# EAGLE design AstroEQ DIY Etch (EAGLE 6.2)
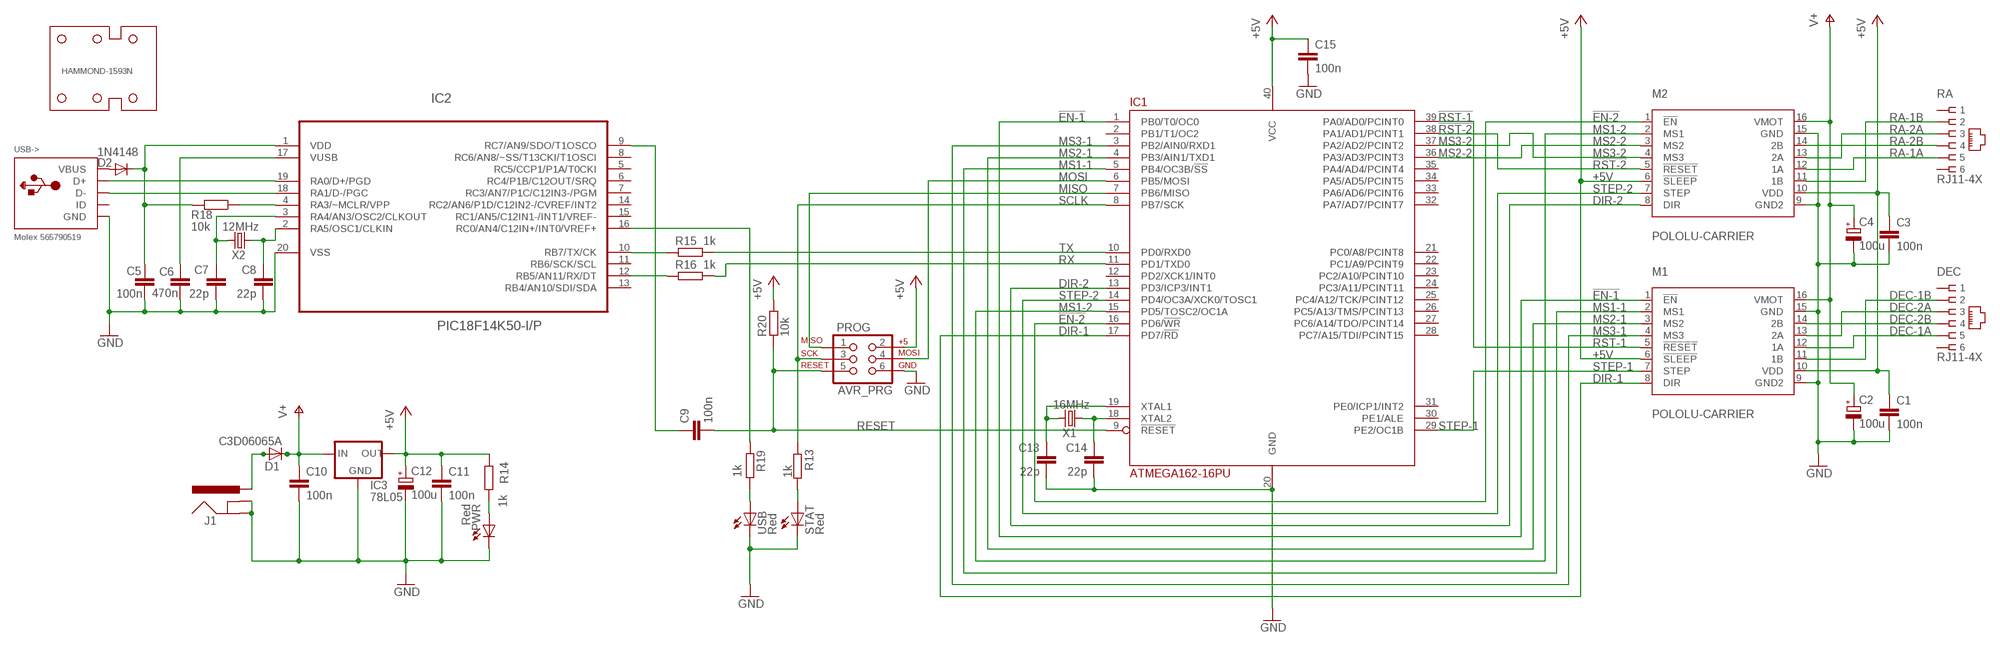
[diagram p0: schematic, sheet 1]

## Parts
C1  100n  C-EU025-024X044  [C025-024X044]
C2  100u  CPOL-EUE2.5-7  [E2,5-7]
C3  100n  C-EU025-024X044  [C025-024X044]
C4  100u  CPOL-EUE2.5-7  [E2,5-7]
C5  100n  C-EU025-024X044  [C025-024X044]
C6  470n  C-EU025-024X044  [C025-024X044]
C7  22p  C-EU025-024X044  [C025-024X044]
C8  22p  C-EU025-024X044  [C025-024X044]
C9  100n  C-EU025-024X044  [C025-024X044]
C10  100n  C-EU025-024X044  [C025-024X044]
C11  100n  C-EU025-024X044  [C025-024X044]
C12  100u  CPOL-EUE2.5-7  [E2,5-7]
C13  22p  C-EU025-024X044  [C025-024X044]
C14  22p  C-EU025-024X044  [C025-024X044]
C15  100n  C-EU025-024X044  [C025-024X044]
D1  C3D06065A  MUR820  [C221B1A]
D2  1N4148  DIODE1N4148  [DIODE-1N4148]
DEC  RJ11-4X  [RJ11-NO_SHIELD]
HAMMOND-1593N  HAMMOND-1593N  [HAMMOND-1593N]
IC1  ATMEGA162-16PU  [DIL40]
IC2  PIC18F14K50-I/P  [DIL20]
IC3  78L05  V_REG_78XXTO-92  [TO-92]
J1  POWER_JACKPTH  [POWER_JACK_PTH]
M1  POLOLU-CARRIER  A4983CARRIER  [DIP16-W]
M2  POLOLU-CARRIER  A4983CARRIER  [DIP16-W]
PROG  AVR_PRG  AVR_SPI_PRG_6PTH  [2X3]
PWR  Red  LED3MM  [LED3MM]
R13  1k  R-EU_0204/7  [0204/7]
R14  1k  R-EU_0204/7  [0204/7]
R15  1k  R-EU_0204/7  [0204/7]
R16  1k  R-EU_0204/7  [0204/7]
R18  10k  R-EU_0204/7  [0204/7]
R19  1k  R-EU_0204/7  [0204/7]
R20  10k  R-EU_0204/7  [0204/7]
RA  RJ11-4X  [RJ11-NO_SHIELD]
STAT  Red  LED3MM  [LED3MM]
USB  Red  LED3MM  [LED3MM]
USB->  Molex 565790519  USBMOLEX  [USB-MINIB-THM-MOLEX]
X1  16MHz  CRYSTALHC49US  [HC49US]
X2  12MHz  CRYSTALHC49US  [HC49US]

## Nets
!EN-1: IC1.1(PB0/T0/OC0) M1.1(!EN)
!EN-2: IC1.16(PD6/!WR) M2.1(!EN)
!RST-1: IC1.39(PA0/AD0/PCINT0) M1.5(!RESET)
!RST-2: IC1.38(PA1/AD1/PCINT1) M2.5(!RESET)
+5V: C1.1 C3.1 C11.1 C12.+ C15.1 IC1.40(VCC) IC3.1(OUT) M1.6(!SLEEP) M1.10(VDD) M2.6(!SLEEP) M2.10(VDD) PROG.2 R14.1 R20.2
AVROSC1: C13.1 IC1.19(XTAL1) X1.2
AVROSC2: C14.1 IC1.18(XTAL2) X1.1
D+: IC2.19(RA0/D+/PGD) USB->.D+
D-: IC2.18(RA1/D-/PGC) USB->.D-
DEC-1A: DEC.5 M1.12(1A)
DEC-1B: DEC.2 M1.11(1B)
DEC-2A: DEC.3 M1.13(2A)
DEC-2B: DEC.4 M1.14(2B)
DIR-1: IC1.17(PD7/!RD) M1.8(DIR)
DIR-2: IC1.13(PD3/ICP3/INT1) M2.8(DIR)
DTR: C9.1 IC2.9(RC7/AN9/SDO/T1OSCO)
GND: C1.2 C2.- C3.2 C4.- C5.2 C6.1 C7.2 C8.2 C10.2 C11.2 C12.- C13.2 C14.2 C15.2 IC1.20(GND) IC2.20(VSS) IC3.2(GND) J1.GND J1.GNDBREAK M1.9(GND2) M1.15(GND) M2.9(GND2) M2.15(GND) PROG.6 PWR.K(C) STAT.K(C) USB->.GND USB->.GND1(GND) USB->.GND4(GND) USB.K(C)
MCLR: IC2.4(RA3/~MCLR/VPP) R18.1
MISO: IC1.7(PB6/MISO) PROG.1
MOSI: IC1.6(PB5/MOSI) PROG.4
MS1-1: IC1.5(PB4/OC3B/!SS) M1.2(MS1)
MS1-2: IC1.15(PD5/TOSC2/OC1A) M2.2(MS1)
MS2-1: IC1.4(PB3/AIN1/TXD1) M1.3(MS2)
MS2-2: IC1.36(PA3/AD3/PCINT3) M2.3(MS2)
MS3-1: IC1.3(PB2/AIN0/RXD1) M1.4(MS3)
MS3-2: IC1.37(PA2/AD2/PCINT2) M2.4(MS3)
PWRLED: PWR.A R14.2
RA-1A: M2.12(1A) RA.5
RA-1B: M2.11(1B) RA.2
RA-2A: M2.13(2A) RA.3
RA-2B: M2.14(2B) RA.4
RESET: C9.2 IC1.9(!RESET) PROG.5 R20.1
RX: IC1.11(PD1/TXD0) R16.1
RX(USB): IC2.12(RB5/AN11/RX/DT) R16.2
SCLK: IC1.8(PB7/SCK) PROG.3 R13.1
STATLED: R13.2 STAT.A
STEP-1: IC1.29(PE2/OC1B) M1.7(STEP)
STEP-2: IC1.14(PD4/OC3A/XCK0/TOSC1) M2.7(STEP)
TX: IC1.10(PD0/RXD0) R15.1
TX(USB): IC2.10(RB7/TX/CK) R15.2
USBLED: R19.1 USB.A
USBOSC1: C8.1 IC2.2(RA5/OSC1/CLKIN) X2.1
USBOSC2: C7.1 IC2.3(RA4/AN3/OSC2/CLKOUT) X2.2
USBSTAT: IC2.16(RC0/AN4/C12IN+/INT0/VREF+) R19.2
V+: C2.+ C4.+ C10.1 D1.C IC3.3(IN) M1.16(VMOT) M2.16(VMOT)
VBUS: D2.A USB->.VBUS
VIN: D1.A J1.PWR
VPIC: C5.1 D2.C IC2.1(VDD) R18.2
VUSB: C6.2 IC2.17(VUSB)
Unconnected: DEC.1 DEC.6 IC1.2(PB1/T1/OC2) IC1.12(PD2/XCK1/INT0) IC1.21(PC0/A8/PCINT8) IC1.22(PC1/A9/PCINT9) IC1.23(PC2/A10/PCINT10) IC1.24(PC3/A11/PCINT11) IC1.25(PC4/A12/TCK/PCINT12) IC1.26(PC5/A13/TMS/PCINT13) IC1.27(PC6/A14/TDO/PCINT14) IC1.28(PC7/A15/TDI/PCINT15) IC1.30(PE1/ALE) IC1.31(PE0/ICP1/INT2) IC1.32(PA7/AD7/PCINT7) IC1.33(PA6/AD6/PCINT6) IC1.34(PA5/AD5/PCINT5) IC1.35(PA4/AD4/PCINT4) IC2.5(RC5/CCP1/P1A/T0CKI) IC2.6(RC4/P1B/C12OUT/SRQ) IC2.7(RC3/AN7/P1C/C12IN3-/PGM) IC2.8(RC6/AN8/~SS/T13CKI/T1OSCI) IC2.11(RB6/SCK/SCL) IC2.13(RB4/AN10/SDI/SDA) IC2.14(RC2/AN6/P1D/C12IN2-/CVREF/INT2) IC2.15(RC1/AN5/C12IN1-/INT1/VREF-) RA.1 RA.6 USB->.ID

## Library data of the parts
C1 C3 C5 C9-C11 C15 = resistor:C-EU: CAPACITOR, European symbol; MF: AVX; MPN: SR205C104KAR; OC_FARNELL: 1100367
C2 C4 C12 = resistor:CPOL-EU: POLARIZED CAPACITOR, European symbol; MF: MULTICOMP; MPN: MCGPR25V107M6.3X11; OC_FARNELL: 9451188
C6 = rcl:C-EU: CAPACITOR, European symbol; MF: KEMET; MPN: C320C474M5U5TA; OC_FARNELL: 1457660
C7 C8 C13 C14 = rcl:C-EU: CAPACITOR, European symbol; MF: AVX; MPN: SR151A220JAR; OC_FARNELL: 1100369
D1 = diode:MUR820: DIODE; MF: CREE; MPN: C3D06065A; OC_FARNELL: 1864928
D2 = SparkFun:DIODE: Diode; MF: MULTICOMP; MPN: 1N4148.; OC_FARNELL: 9565124
DEC RA = con-tycoelectronics:RJ11: CORCOM Modular RJ Jacks No Shield Source: www.tycoelectronics.com .. ENG_DS_1654001_1099_RJ_L_0507.pdf; MF: MOLEX; MPN: 95501-2641; OC_FARNELL: 1560166; OC_NEWARK: 19R7022
HAMMOND-1593N = holes:HAMMOND-1593N; MF: HAMMOND; MPN: 1593NBK; OC_FARNELL: 9287566
IC1 = atmel:ATMEGA162: 8-bit RISC MICROCONTROLLER 16K Bytes internal flash program memory 1K Bytes internal SRAM Upto 64K Bytes optional external memory space 512 Bytes EEPROM Two 8-bit timers Two 16-bit timers Dual programmable serial USARTs Master/Slave serial SPI interface Source: ATMEGA162_DIP40.lbr; MF: ATMEL; MPN: ATMEGA162-16PU; OC_FARNELL: 9171169
IC2 = microchip:PIC18F14K50-I/P: USB Flash Microcontrollers; MF: MICROCHIP; MPN: PIC18F14K50-I/P; OC_FARNELL: 1648501; OC_NEWARK: 77M3103; PACKAGE: DIP-20; SUPPLIER: Microchip
IC3 = SparkFun:V_REG_78XX: Voltage Regulator Standard 7805 5V regulator. IGO (Input Ground Output). Spark Fun Electronics SKU : COM-00107; MF: FAIRCHILD SEMICONDUCTOR; MPN: LM78L05ACZX; OC_FARNELL: 1467367
J1 = SparkFun:POWER_JACK: Power Jack This is the standard 5.5mm barrel jack for power. The PTH is the most common, proven, reliable, footprint. All others are experimental. The Slot footprint only works if the mill layer is transmitted to the PCB fab house so be warned. Spark Fun Electronics SKU : PRT-00119. Mating wall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; MF: MULTICOMP; MPN: MJ-179PH; OC_FARNELL: 1737246
M1 M2 = A4983Carrier:A4983CARRIER; MF: SAMTEC; MPN: CES-116-01-T-S; OC_FARNELL: 1667522
PROG = SparkFun:AVR_SPI_PRG_6: AVR ISP 6 Pin This is the reduced ISP connector for AVR programming. Common on Arduino. This footprint will take up less PCB space and can be used with a 10-pin to 6-pin adapter such as SKU: BOB-08508; MF: TE CONNECTIVITY / AMP; MPN: 826632-3; OC_FARNELL: 3418492
PWR STAT USB = led:LED: LED; MF: KINGBRIGHT; MPN: L-424HDT; OC_FARNELL: 1142499
R13 R14 R19 = rcl:R-EU_: RESISTOR, European symbol; MF: MULTICOMP; MPN: MF12 1K; OC_FARNELL: 9342400
R15 R16 = SmartPrj:R-EU_: RESISTOR, European symbol; MF: MULTICOMP; MPN: MF12 1K; OC_FARNELL: 9342400
R18 R20 = rcl:R-EU_: RESISTOR, European symbol; MF: MULTICOMP; MPN: MF12 10K; OC_FARNELL: 9342419
USB-> = adafruit:USB: USB Connectors USBMINIB - Surface Mount Female Mini-B USB Connector 4UConnector: 06564 By microbuilder.eu Thru-hole RA Female Mini-B USB Connector 4UConnector: 18732 By ladyada.net; MF: MOLEX; MPN: 565790519; OC_FARNELL: 1125347
X1 = SparkFun:CRYSTAL: Crystals; MF: TXC; MPN: 9B-16.000MEEJ-B; OC_FARNELL: 1842217
X2 = SparkFun:CRYSTAL: Crystals; MF: TXC; MPN: 9B-12.000MAAJ-B; OC_FARNELL: 1842203

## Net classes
1 power: width 0.61 mm, drill 0.711 mm, clearance 0.203 mm
2 gnd: width 0.305 mm, drill 0.711 mm, clearance 0.203 mm
3 usbvcc: width 0.508 mm, drill 0.711 mm, clearance 0.203 mm

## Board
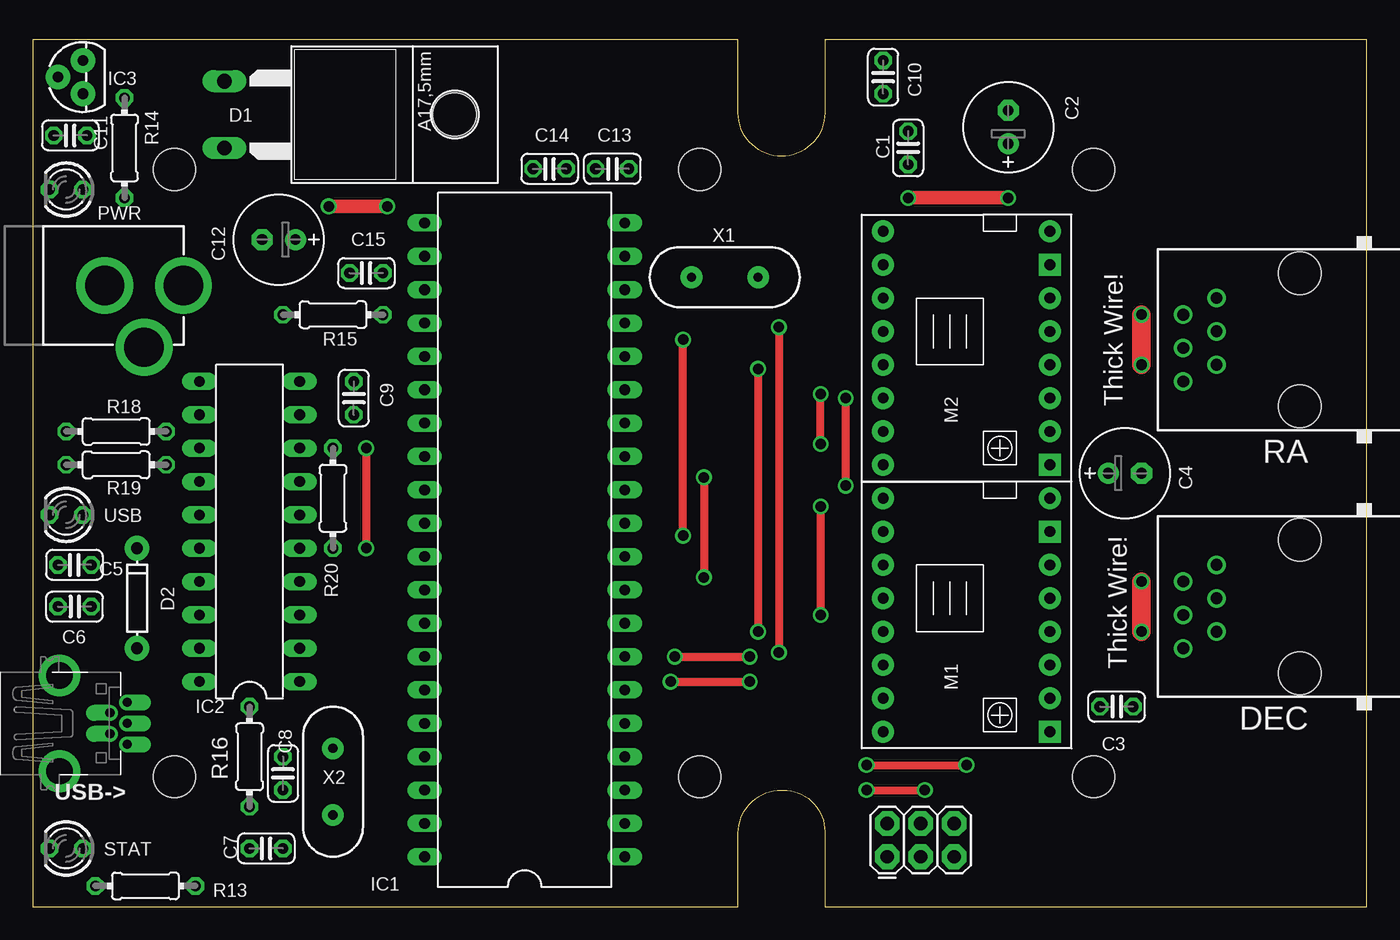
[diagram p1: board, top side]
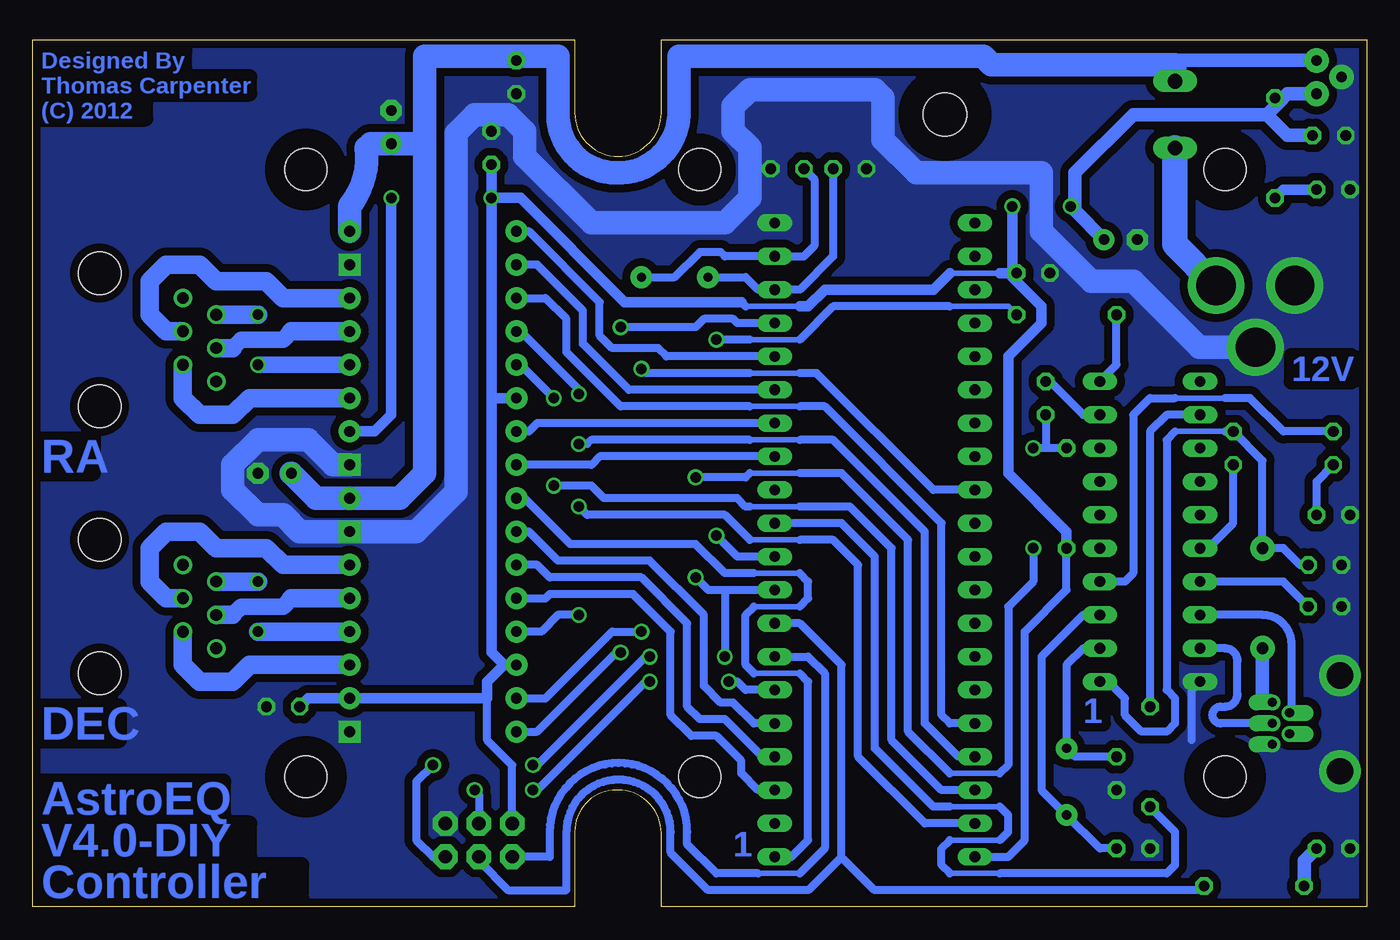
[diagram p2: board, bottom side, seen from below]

Size 101.6 x 66.04 mm. Coordinates in mm from the lower left corner, seen from the top.
Outline: 57.02,8.89 57.15,8.89
Copper layers (1*16): Top 0.035mm / dielectric 1.5mm / Bottom 0.035mm
Design rules: minimum track width 10mil, minimum drill 24mil, track to track 8mil, track to pad 8mil, pad to pad 8mil, via to via 8mil, smd to smd 8mil, copper to edge 8mil, drill to drill 8mil, minimum pad ring 10mil, minimum via ring 8mil, stop-mask expansion 4mil, vias tented up to drill 0mil, thermal gap 10mil
tKeepout: area 78.3,7.4 to 83.3,12.4; area 78.3,53.6 to 83.3,58.6; area 48.3,7.4 to 53.3,12.4; area 8.3,7.4 to 13.3,12.4; area 48.3,53.6 to 53.3,58.6; area 8.3,53.6 to 13.3,58.6
bKeepout: area 78.3,7.4 to 83.3,12.4; area 78.3,53.6 to 83.3,58.6; area 48.3,7.4 to 53.3,12.4; area 8.3,7.4 to 13.3,12.4; area 48.3,53.6 to 53.3,58.6; area 8.3,53.6 to 13.3,58.6
bRestrict: area 78.3,53.6 to 83.3,58.6; area 78.3,7.4 to 83.3,12.4; area 8.3,7.4 to 13.3,12.4; area 8.3,53.6 to 13.3,58.6; 2 lines

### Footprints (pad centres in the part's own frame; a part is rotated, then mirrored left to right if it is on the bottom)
C025-024X044 = drill 0.813 octagon: 1 -1.27,0; 2 1.27,0
E2,5-7 = drill 0.813 pad 1.6: + -1.27,0 | drill 0.813 pad 1.6 octagon: - 1.27,0
C221B1A = drill 1.118 long: A 2.54,-6.35; C -2.54,-6.35 | hole 3.302: 0,11.176
DIODE-1N4148 = drill 0.9 pad 1.88: A -3.81,0; C 3.81,0
RJ11-NO_SHIELD = drill 0.9 pad 1.4: 1 -3.175,8.89; 2 -1.905,6.35; 3 -0.635,8.89; 4 0.635,6.35; 5 1.905,8.89; 6 3.175,6.35 | hole 3.251: -5.08,0; 5.08,0
HAMMOND-1593N = hole 3.2: 10.795,9.906; 10.795,56.134; 50.8,9.906; 50.8,56.134; 80.797,9.906; 80.797,56.134
DIL40 = drill 0.813 long: 1 -24.13,-7.62; 2 -21.59,-7.62; 3 -19.05,-7.62; 4 -16.51,-7.62; 5 -13.97,-7.62; 6 -11.43,-7.62; 7 -8.89,-7.62; 8 -6.35,-7.62; 9 -3.81,-7.62; 10 -1.27,-7.62; 11 1.27,-7.62; 12 3.81,-7.62; 13 6.35,-7.62; 14 8.89,-7.62; 15 11.43,-7.62; 16 13.97,-7.62; 17 16.51,-7.62; 18 19.05,-7.62; 19 21.59,-7.62; 20 24.13,-7.62; 21 24.13,7.62; 22 21.59,7.62; 23 19.05,7.62; 24 16.51,7.62; 25 13.97,7.62; 26 11.43,7.62; 27 8.89,7.62; 28 6.35,7.62; 29 3.81,7.62; 30 1.27,7.62; 31 -1.27,7.62; 32 -3.81,7.62; 33 -6.35,7.62; 34 -8.89,7.62; 35 -11.43,7.62; 36 -13.97,7.62; 37 -16.51,7.62; 38 -19.05,7.62; 39 -21.59,7.62; 40 -24.13,7.62
DIL20 = drill 0.813 long: 1 -3.81,11.43; 2 -3.81,8.89; 3 -3.81,6.35; 4 -3.81,3.81; 5 -3.81,1.27; 6 -3.81,-1.27; 7 -3.81,-3.81; 8 -3.81,-6.35; 9 -3.81,-8.89; 10 -3.81,-11.43; 11 3.81,-11.43; 12 3.81,-8.89; 13 3.81,-6.35; 14 3.81,-3.81; 15 3.81,-1.27; 16 3.81,1.27; 17 3.81,3.81; 18 3.81,6.35; 19 3.81,8.89; 20 3.81,11.43
TO-92 = drill 0.813 pad 1.88: 1 -1.27,0; 2 0,1.905; 3 1.27,0
POWER_JACK_PTH = drill 2.997 pad 4.318: GND 0,7.7; GNDBREAK 4.7,10.7; PWR 0,13.7
DIP16-W = drill 0.813 pad 1.676: 1 -8.89,-6.35; 2 -6.35,-6.35; 3 -3.81,-6.35; 4 -1.27,-6.35; 5 1.27,-6.35; 6 3.81,-6.35; 7 6.35,-6.35; 8 8.89,-6.35; 10 6.35,6.35; 11 3.81,6.35; 12 1.27,6.35; 13 -1.27,6.35; 14 -3.81,6.35; 16 -8.89,6.35 | drill 0.813 pad 1.676 square: 9 8.89,6.35; 15 -6.35,6.35
2X3 = drill 1.016 pad 1.88 octagon: 1 0,0; 2 0,2.54; 3 2.54,0; 4 2.54,2.54; 5 5.08,0; 6 5.08,2.54
LED3MM = drill 0.813 octagon: A -1.27,0; K 1.27,0
0204/7 = drill 0.813 octagon: 1 -3.81,0; 2 3.81,0
USB-MINIB-THM-MOLEX = drill 0.7 offset: D+ 0,9.72; D- -0.8,8.42; GND 1.6,9.72; ID 0.8,8.42; VBUS -1.6,9.72 | drill 2 pad 3.175: GND1 -3.65,4.57; GND4 3.65,4.57
HC49US = drill 0.7 pad 1.651: 1 -2.54,0; 2 2.54,0

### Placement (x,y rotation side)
C1  66.67,57.78 90 top
C2  74.3,59.37 90 top
C3  82.55,15.24 0 top
C4  83.19,33.02 0 top
C5  3.17,26.04 180 top
C6  3.17,22.86 0 top
C7  17.78,4.45 180 top
C8  19.05,10.16 270 top
C9  24.45,38.73 270 top
C10  64.77,63.18 270 top
C11  2.86,58.74 180 top
C12  18.73,50.8 180 top
C13  44.13,56.2 0 top
C14  39.37,56.2 180 top
C15  25.4,48.26 180 top
D1  20.95,60.33 270 top
D2  7.94,23.5 90 top
DEC  96.52,22.86 90 top
HAMMOND-1593N  0,0 0 top
IC1  37.47,27.94 90 top
IC2  16.51,28.57 180 top
IC3  3.81,63.18 90 top
J1  -2.22,47.31 270 top
M1  71.12,22.23 270 top
M2  71.12,42.55 270 top
PROG  65.09,3.81 0 top
PWR  2.54,54.61 180 top
R13  8.57,1.59 180 top
R14  6.99,57.78 270 top
R15  22.86,45.09 180 top
R16  16.51,11.43 90 top
R18  6.35,36.2 0 top
R19  6.35,33.66 0 top
R20  22.86,31.11 270 top
RA  96.52,43.18 90 top
STAT  2.54,4.45 180 top
USB  2.54,29.84 180 top
USB->  -2.54,13.97 270 top
X1  52.7,47.94 0 top
X2  22.86,9.53 270 top

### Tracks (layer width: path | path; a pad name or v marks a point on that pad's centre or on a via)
!EN-1
  Bottom 0.406: 43.18,17.78 46.67,17.78 | 46.67,22.86 43.18,22.86 | 43.18,25.4 46.67,25.4
  Bottom 0.61: IC1.1 43.81,3.81 42.55,5.08 42.55,17.14 43.18,17.78 | 46.67,17.78 47.31,18.41 47.31,22.23 46.67,22.86 | 43.18,22.86 42.55,23.5 42.55,24.77 43.18,25.4 | 46.67,25.4 48.9,25.4 51.12,27.62 60.64,27.62 64.14,31.11 M1.1
!EN-2
  Bottom 0.61: IC1.16 53.34,41.91 53.98,42.55 57.47,42.55 58.42,43.5 58.42,46.04 63.82,51.44 M2.1
!RST-1  (via drill 0.8)
  Top 0.61: v60.01,30.48 v60.01,22.23
  Bottom 0.406: 43.18,27.94 46.99,27.94
  Bottom 0.61: IC1.39 33.66,6.35 38.73,11.43 38.73,26.04 40.64,27.94 43.18,27.94 | 46.99,27.94 48.9,29.84 59.37,29.84 v60.01,30.48 | v60.01,22.23 61.59,22.23 62.87,20.95 M1.5
!RST-2  (via drill 0.8)
  Top 0.61: v61.91,38.73 v61.91,32.07
  Bottom 0.406: 43.18,30.48 46.99,30.48
  Bottom 0.61: M2.5 64.45,41.27 v61.91,38.73 | IC1.38 32.38,8.89 36.2,12.7 36.2,27.3 39.37,30.48 43.18,30.48 | 46.99,30.48 47.31,30.48 47.94,31.11 58.1,31.11 59.05,32.07 v61.91,32.07
+5V  (via drill 0.8)
  Top 1.016: v66.67,53.98 v74.3,53.98 | v22.54,53.34 v26.99,53.34
  Bottom 0.406: 27.94,48.26 31.75,48.26 | 43.18,45.72 47.31,45.72
  Bottom 0.61: IC1.40 27.3,3.81 26.04,5.08 26.04,20.95 22.86,24.13 R20.2 | 47.31,45.72 47.62,46.04 | PROG.2 65.09,10.79 66.99,12.7 66.99,15.88
  Bottom 0.813: C3.1 80.64,15.88 M1.10 66.99,15.88 66.99,17.14 65.72,18.41 | M2.10 75.56,36.2 74.3,37.47 v74.3,53.98 | M1.6 65.72,18.41 | v66.67,53.98 C1.1 | R20.2 22.86,28.57 27.3,33.02 27.3,41.91 24.77,44.45 24.77,45.72 26.99,47.94 26.99,48.26 | C15.1 26.99,48.26 | 26.99,48.26 27.94,48.26 | 31.75,48.26 33.02,46.99 41.27,46.99 42.55,45.72 43.18,45.72 | 47.62,46.04 56.52,46.04 64.45,53.98 v66.67,53.98 | 22.23,53.66 22.23,53.34 v22.54,53.34 | v26.99,53.34 26.99,48.26 | M2.6 66.67,38.73 | v66.67,53.98 66.67,38.73 | 66.67,38.73 66.67,19.37 65.72,18.41
  Bottom 1.016: IC3.1 6.03,61.91 6.67,61.28 | 6.67,61.28 7.62,60.33 | 7.62,60.33 17.78,60.33 22.23,55.88 22.23,53.66 22.23,53.02 C12.+ | R14.1 6.67,61.28 | C11.1 6.03,58.74 7.62,60.33
AVROSC1
  Bottom 0.61: C13.1 42.07,55.4 42.07,50.32 42.86,49.53 IC1.19 48.9,49.53 49.21,49.85 50.8,49.85 52.7,47.94 X1.2
AVROSC2
  Bottom 0.61: C14.1 40.64,49.53 43.18,46.99 IC1.18 46.35,46.99 47.31,47.94 X1.1
D+
  Bottom 0.61: USB->.D+ 11.11,13.97 arc90 11.75,14.61 arc90 11.11,15.24 10.79,15.24 arc-90 9.84,16.19 9.84,18.73 arc-90 10.79,19.68 IC2.19
D-
  Bottom 0.61: USB->.D- 5.71,14.77 5.71,20 arc-90 7.94,22.23 IC2.18
DEC-1A  (via drill 0.8)
  Top 1.422: v84.45,20.95 v84.45,24.77
  Bottom 1.422: v84.45,24.77 DEC.5 | v84.45,20.95 M1.12
DEC-1B
  Bottom 1.422: M1.11 85.09,18.41 86.36,17.14 88.9,17.14 90.17,18.41 DEC.2
DEC-2A
  Bottom 1.27: 81.92,23.5 82.55,22.86 85.72,22.86 86.36,22.23
  Bottom 1.422: DEC.3 86.36,22.23 | M1.13 81.92,23.5
DEC-2B
  Bottom 1.422: M1.14 82.55,26.04 83.82,27.3 87.63,27.3 88.9,28.57 91.44,28.57 92.71,27.3 92.71,24.77 91.44,23.5 DEC.4
DIR-1  (via drill 0.8)
  Top 0.61: v56.83,44.13 v56.83,19.37
  Bottom 0.61: IC1.17 47.94,44.45 48.26,44.77 50.48,44.77 51.12,44.13 v56.83,44.13 | M1.8 63.18,13.34 57.15,19.37 v56.83,19.37
DIR-2
  Bottom 0.61: IC1.13 58.42,34.29 59.05,33.66 M2.8
DTR
  Bottom 0.61: C9.1 24.13,40.01 21.59,37.47 IC2.9
GND
  Bottom 0.61: 13.34,12.7 13.34,16.51 IC2.20
  Bottom 1.778: J1.GNDBREAK 12.76,42.61 17.78,47.62 20.95,47.62 24.77,51.44 24.77,55.88 34.29,55.88 36.83,58.42 36.83,61.59 37.47,62.23 46.99,62.23 48.26,60.96 48.26,59.05 46.99,57.78 46.99,53.98 48.9,52.07 59.05,52.07 64.14,57.15 64.14,59.05 65.41,60.33 67.94,60.33 69.37,58.9 69.37,31.59 72.39,28.57 M1.15 81.28,28.57 82.55,29.84 84.45,29.84 86.36,31.75 86.36,33.66 84.45,35.56 80.64,35.56 78.74,33.66 M2.9
  pour Bottom (isolate 0.61, no thermals): -1.27,66.99 102.62,66.99 102.62,-0.95 -1.27,-0.95
MCLR
  Bottom 0.406: 10.79,38.73 14.61,38.73
  Bottom 0.61: R18.1 6.35,36.2 8.89,38.73 10.79,38.73 | IC2.4 18.41,24.77 17.78,25.4 17.78,37.47 16.51,38.73 14.61,38.73
MISO
  Bottom 0.406: 43.18,2.54 46.35,2.54
  Bottom 0.61: IC1.7 42.55,19.05 41.27,17.78 41.27,4.45 43.18,2.54 | 46.35,2.54 49.53,2.54 51.75,4.76 51.75,5.71 arc-180 62.23,5.71 62.23,3.81 PROG.1
MOSI  (via drill 0.8)
  Top 0.61: v48.58,17.14 v54.61,17.14 | v63.5,8.89 v67.94,8.89
  Bottom 0.61: IC1.6 47.31,16.51 47.94,17.14 v48.58,17.14 | v54.61,17.14 54.93,17.14 63.18,8.89 v63.5,8.89 | v67.94,8.89 67.63,8.57 PROG.4
MS1-1
  Bottom 0.61: IC1.5 46.67,13.97 48.26,15.56 49.21,15.56 50.48,16.83 50.48,22.23 54.61,26.35 61.59,26.35 63.82,28.57 M1.2
MS1-2
  Bottom 0.61: IC1.15 56.2,39.37 59.69,42.86 59.69,45.4 63.18,48.9 M2.2
MS2-1
  Bottom 0.61: IC1.4 46.04,11.43 48.9,14.29 50.8,14.29 51.75,15.24 51.75,21.59 55.24,25.08 62.23,25.08 63.18,26.04 M1.3
MS2-2
  Bottom 0.406: 43.18,38.1 46.99,38.1
  Bottom 0.61: M2.3 62.55,46.35 60.96,44.77 60.96,42.23 56.83,38.1 46.99,38.1 | IC1.36 31.75,13.97 32.38,14.61 32.38,29.21 41.27,38.1 43.18,38.1
MS3-1
  Bottom 0.61: IC1.3 46.35,8.89 47.62,10.16 47.62,11.11 49.53,13.02 51.44,13.02 53.02,14.61 53.02,20.95 55.88,23.81 62.23,23.81 62.55,23.5 M1.4
MS3-2  (via drill 0.8)
  Top 0.61: v60.01,35.24 v60.01,39.05
  Bottom 0.406: 43.18,35.56 46.99,35.56
  Bottom 0.61: M2.4 64.45,43.81 60.01,39.37 v60.01,39.05 | IC1.37 31.11,11.43 33.66,13.97 33.66,28.57 40.64,35.56 43.18,35.56 | 46.99,35.56 59.05,35.56 59.37,35.24 v60.01,35.24
PWRLED
  Bottom 0.813: R14.2 6.35,54.61 PWR.A
RA-1A  (via drill 0.8)
  Top 1.422: v84.45,41.27 v84.45,45.09
  Bottom 1.27: M2.12 v84.45,41.27
  Bottom 1.422: v84.45,45.09 RA.5
RA-1B
  Bottom 1.422: M2.11 85.09,38.73 86.36,37.47 88.9,37.47 90.17,38.73 RA.2
RA-2A
  Bottom 1.27: 86.36,42.55 85.72,43.18 82.55,43.18 81.92,43.81
  Bottom 1.422: RA.3 86.36,42.55 | 81.92,43.81 M2.13
RA-2B
  Bottom 1.422: RA.4 91.44,43.81 92.71,45.09 92.71,47.62 91.44,48.9 88.9,48.9 87.63,47.62 83.82,47.62 82.55,46.35 M2.14
RESET  (via drill 0.8)
  Top 0.61: v25.4,34.92 v25.4,27.3 | v51.12,32.7 v51.12,25.08 | v48.9,19.05 v54.61,19.05 | v63.5,10.79 v71.12,10.79
  Bottom 0.406: 27.94,10.16 31.75,10.16 | 43.18,33.02 46.99,33.02
  Bottom 0.61: R20.1 24.45,34.92 | C9.2 24.45,34.92 | 24.45,34.92 v25.4,34.92 | v25.4,27.3 25.4,24.77 27.3,22.86 27.3,10.79 27.94,10.16 | 31.75,10.16 34.92,13.34 34.92,27.94 40.01,33.02 43.18,33.02 | 46.99,33.02 47.31,32.7 v51.12,32.7 | v51.12,25.08 50.16,24.13 48.9,24.13 | 48.9,24.13 IC1.9 | 48.9,24.13 v48.9,19.05 | v54.61,19.05 54.93,19.05 63.18,10.79 v63.5,10.79 | v71.12,10.79 72.39,9.53 72.39,5.08 71.12,3.81 PROG.5
RX
  Bottom 0.406: 27.94,2.54 31.75,2.54 | 31.75,5.08 27.94,5.08 | 27.94,7.62 31.75,7.62
  Bottom 0.61: R16.1 14.61,5.71 14.61,3.17 15.24,2.54 27.94,2.54 | 31.75,2.54 32.38,3.17 32.38,4.45 31.75,5.08 | 27.94,5.08 27.3,5.71 27.3,6.99 27.94,7.62 | 31.75,7.62 33.02,7.62 37.47,12.06 37.47,26.67 40.01,29.21 IC1.11
RX(USB)
  Bottom 0.61: IC2.12 15.24,37.47 16.51,36.2 R16.2
SCLK
  Bottom 0.61: R13.1 12.7,1.27 37.49,1.27 40.01,3.79 | 40.01,3.79 40.01,18.41 43.18,21.59 IC1.8 | 40.01,3.79 42.52,1.27 50.16,1.27 53.02,4.13 53.02,5.71 arc-180 60.96,5.71 60.96,1.27 65.41,1.27 67.63,3.49 PROG.3
STATLED
  Bottom 1.016: STAT.A 4.76,3.49 R13.2
STEP-1  (via drill 0.8)
  Top 0.61: v55.24,40.96 v55.24,20.95
  Bottom 0.406: 43.18,40.64 46.99,40.64
  Bottom 0.61: IC1.29 33.02,31.75 41.91,40.64 43.18,40.64 | 46.99,40.64 54.93,40.64 v55.24,40.96 | M1.7 62.55,15.88 57.47,20.95 v55.24,20.95
STEP-2
  Bottom 0.61: IC1.14 63.18,36.83 63.82,36.2 M2.7
TX  (via drill 0.8)
  Top 0.61: v49.53,28.26 v49.53,43.18
  Bottom 0.406: R15.1 27.3,45.72 31.75,45.72 | 43.18,43.18 46.99,43.18
  Bottom 0.61: 31.75,45.72 40.64,45.72 43.18,43.18 | 46.99,43.18 v49.53,43.18 | IC1.10 47.94,26.67 v49.53,28.26
TX(USB)
  Bottom 0.61: IC2.10 19.05,41.27 R15.2
USBLED
  Bottom 0.61: USB.A 3.81,32.38 R19.1
USBOSC1
  Bottom 0.61: IC2.2 21.59,19.68 22.86,18.41 X2.1 22.23,11.43 C8.1
USBOSC2
  Bottom 0.61: IC2.3 21.59,22.23 24.77,19.05 24.77,8.89 X2.2 20.32,4.45 C7.1
USBSTAT
  Bottom 0.61: IC2.16 12.06,27.3 10.16,29.21 R19.2
V+
  Bottom 0.406: 14.61,63.5 D1.C
  Bottom 0.61: C10.1 64.77,64.77 | 14.61,63.5 14.61,64.45 14.29,64.45
  Bottom 1.016: IC3.3 14.29,64.45
  Bottom 1.778: C4.+ 80.01,31.11 M1.16 73.66,31.11 71.75,33.02 71.75,58.1 | 71.75,58.1 71.75,64.77 64.77,64.77 61.59,64.77 61.59,60.33 arc-90 57.15,55.88 arc-90 52.39,60.33 52.39,64.77 29.21,64.77 28.57,64.14 14.61,64.14 14.61,63.5 | M2.16 77.47,53.34 arc-45 76.2,57.78 75.88,58.1 C2.+ 71.75,58.1
VBUS
  Bottom 1.016: USB->.VBUS 7.94,15.57 D2.A
VIN
  Bottom 1.93: J1.PWR 14.61,50.44 D1.A
VPIC
  Bottom 0.406: 10.79,36.2 14.61,36.2
  Bottom 0.61: 10.79,36.2 R18.2 7.94,33.97 D2.C 6.35,27.3 5.08,26.04 C5.1 | 14.61,36.2 15.24,35.56 15.24,16.51 14.61,15.88 14.61,13.97 15.24,13.34 17.14,13.34 18.41,14.61 18.41,15.88 19.68,17.14 IC2.1
VUSB
  Bottom 0.61: C6.2 6.35,24.77 IC2.17

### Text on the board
Bottom: Designed By | Thomas Carpenter | (C) 2012 | 12V | RA | 1 | DEC | AstroEQ | 1 | V4.0-DIY | Controller
tNames: Thick Wire! | Thick Wire!
Reference: This board design is for those who choose to etch the board at home. | Top Layer not used for DIY Board | Use single-sided copper clad board. Preferably 1oz copper and 1.2mm thick (1.6mm acceptable) | Route RED traces with wires after home Etching. | When printing silkscreen on paper, only Tnames and Tvalues (and Dimension) layers should be visible. | If using 1.6mm, area around USB connector needs to be thinned down to 1.2mm thick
